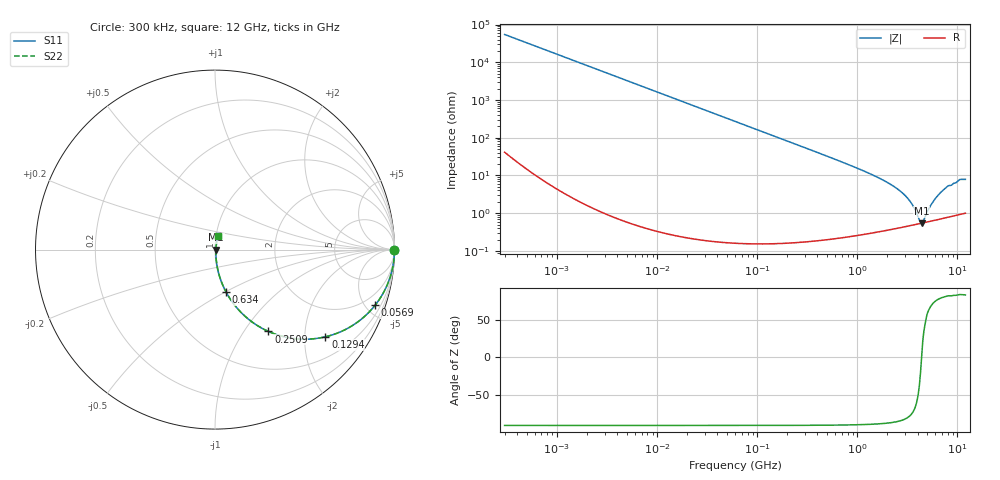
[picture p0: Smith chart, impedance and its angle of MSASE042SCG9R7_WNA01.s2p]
! MSASE042SCG9R7_WNA01  S-PARAMETER MODEL  ( General Type )
! Model Generated by TAIYO YUDEN Corporation (http://www.ty-top.com)
! Version 1.0
! TAIYO YUDEN Control No. 130801
! Copyright(c) 2013 TAIYO YUDEN CO.,LTD. All Rights Reserved.
! Product Description (link to TY-COMPAS)
! https://ds.yuden.co.jp/TYCOMPAS/or/detail?pn=MSASE042SCG9R7BWNA01&u=M
! Products Name : Multilayer Ceramic Capacitors
! Characteristics :
!  Capacitance : 9.7 pF , Rated Voltage : 16V , TCC : CG / C0G
!  Case Size : 0.4 x 0.2 / 0.016 x 0.008 [mm/inch] , Thickness : 0.2 / 0.008 [mm/inch]
!  (Conditions: Temperature = 25 degC , DC Bias Current/Voltage = 0A / 0V)
! External Node Assignments :
!  1  o---| |---o  2
! GND o---------o GND
! Frequency Range : 0.3MHz  -  12000MHz  [ 401 STEP ]
# MHz S RI R 50
! Freq[MHz].  S11 Real  S11 Imag  S21 Real  S21 Imag  S12 Real  S12 Imag  S22 Real  S22 Imag
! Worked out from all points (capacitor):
!   401 points, 300 kHz to 12 GHz, reference 50 ohm
!   read as one part in series: C = 9.72 pF near 316.3 kHz
!   lowest |Z| = 541 mohm at 4.385 GHz (marker M1)
!   series resonance near 4.381 GHz, so ESL is about 140 pH
!   S11 on the Smith chart (normalised r, x): 300 kHz: open; 56.9 MHz: 1.00, -5.75; 129.4 MHz: 1.00, -2.53; 250.9 MHz: 1.00, -1.30; 634 MHz: 1.00, -0.51; 12 GHz: 1.02, +0.16
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0.3  1 -0.00183  4.74e-06 0.00183  4.74e-06 0.00183  1 -0.00183
1.769972  0.9999 -0.0108  0.000119 0.0108  0.000119 0.0108  0.9999 -0.0108
10.44266  0.9959 -0.0635  0.00406 0.0635  0.00406 0.0635  0.9959 -0.0635
25.70316  0.9759 -0.1532  0.0241 0.1532  0.0241 0.1532  0.9759 -0.1532
56.90376  0.8921 -0.31  0.1079 0.31  0.1079 0.31  0.8921 -0.31
60  0.8815 -0.323  0.1185 0.323  0.1185 0.323  0.8815 -0.323
129.3602  0.6152 -0.4859  0.3848 0.4859  0.3848 0.4859  0.6152 -0.4859
250.8588  0.2979 -0.4561  0.7021 0.4561  0.7021 0.4561  0.2979 -0.4561
353.9943  0.1754 -0.3783  0.8246 0.3783  0.8246 0.3783  0.1754 -0.3783
634.0297  0.0619 -0.2367  0.9381 0.2367  0.9381 0.2367  0.0619 -0.2367
1296.429  0.0159 -0.1131  0.9841 0.1131  0.9841 0.1131  0.0159 -0.1131
2088.533  0.00722 -0.06  0.9928 0.06  0.9928 0.06  0.00722 -0.06
2650.866  0.00559 -0.0389  0.9944 0.0389  0.9944 0.0389  0.00559 -0.0389
3190.978  0.00508 -0.024  0.9949 0.024  0.9949 0.024  0.00508 -0.024
3642.919  0.00504 -0.0139  0.995 0.0139  0.995 0.0139  0.00504 -0.0139
4158.869  0.00524 -0.004  0.9948 0.004  0.9948 0.004  0.00524 -0.004
4385.161  0.00539 8.49e-05  0.9946 -8.49e-05  0.9946 -8.49e-05  0.00539 8.49e-05
4623.766  0.00557 0.00391  0.9944 -0.00391  0.9944 -0.00391  0.00557 0.00391
5715.274  0.00665 0.019  0.9934 -0.019  0.9934 -0.019  0.00665 0.019
7064.448  0.00855 0.0375  0.9914 -0.0375  0.9914 -0.0375  0.00855 0.0375
10511.28  0.0148 0.0752  0.9852 -0.0752  0.9852 -0.0752  0.0148 0.0752
12000  0.0158 0.0761  0.9842 -0.0761  0.9842 -0.0761  0.0158 0.0761
